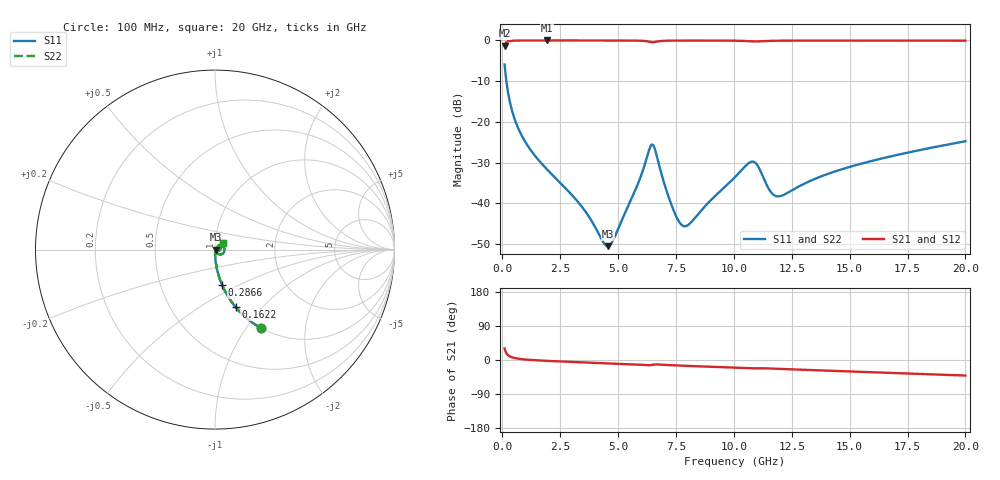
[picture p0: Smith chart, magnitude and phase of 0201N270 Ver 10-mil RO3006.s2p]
# GHz S MA R 50
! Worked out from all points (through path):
!   1601 points, 100 MHz to 20 GHz, reference 50 ohm
!   highest |S21| = -0.02 dB at 1.916 GHz (marker M1); lowest = -1.3 dB at 100 MHz (marker M2)
!   group delay of S21, straight-line fit = 6.12 ps
!   lowest |S11| = -50.5 dB at 4.553 GHz (marker M3), VSWR 1.01, Z = 50.3 - j0.0779 ohm
!   |S11| at or under -10 dB: 176 MHz to end of sweep
!   |S22| runs from -50.5 to -5.9 dB; largest |S21 - S12| = 0
!   S11 on the Smith chart (normalised r, x): 100 MHz: 1.00, -1.17; 162.2 MHz: 1.00, -0.72; 286.6 MHz: 1.00, -0.41; 20 GHz: 1.09, +0.09
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0.1  0.5062 -59.7  0.8616 30.2  0.8616 30.2  0.5062 -59.7
0.1621875  0.3402 -70.3  0.9396 19.6  0.9396 19.6  0.3402 -70.3
0.2865625  0.2002 -78.8  0.9789 11.0  0.9789 11.0  0.2002 -78.8
0.5104375  0.1132 -84.0  0.9926 5.5  0.9926 5.5  0.1132 -84.0
0.8338125  0.06847 -86.7  0.9965 2.3  0.9965 2.3  0.06847 -86.7
1.915875  0.02646 -88.5  0.9979 -2.2  0.9979 -2.2  0.02646 -88.5
3.420812  0.009244 -81.3  0.9975 -6.1  0.9975 -6.1  0.009244 -81.3
4.552625  0.002997 -15.0  0.9969 -8.8  0.9969 -8.8  0.002997 -15.0
4.801375  0.003619 18.4  0.9967 -9.4  0.9967 -9.4  0.003619 18.4
5.709313  0.01383 53.2  0.9939 -11.8  0.9939 -11.8  0.01383 53.2
6.405812  0.05054 10.4  0.9534 -13.6  0.9534 -13.6  0.05054 10.4
6.542625  0.05046 -21.7  0.95 -12.2  0.95 -12.2  0.05046 -21.7
6.741625  0.032 -51.8  0.9751 -11.8  0.9751 -11.8  0.032 -51.8
7.388375  0.008373 -51.3  0.9931 -14.0  0.9931 -14.0  0.008373 -51.3
7.848562  0.005265 -10.4  0.9946 -15.2  0.9946 -15.2  0.005265 -10.4
10.05  0.02108 45.6  0.991 -20.4  0.991 -20.4  0.02108 45.6
10.87087  0.03235 9.7  0.972 -21.9  0.972 -21.9  0.03235 9.7
11.57981  0.01405 -4.3  0.9863 -22.5  0.9863 -22.5  0.01405 -4.3
11.90319  0.01222 14.6  0.99 -23.3  0.99 -23.3  0.01222 14.6
13.37081  0.01932 45.5  0.9936 -26.6  0.9936 -26.6  0.01932 45.5
16.69162  0.03733 47.5  0.9933 -33.8  0.9933 -33.8  0.03733 47.5
20  0.05794 42.9  0.9918 -41.0  0.9918 -41.0  0.05794 42.9
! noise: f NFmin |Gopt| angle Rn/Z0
0.1  0.0005833  0.9266  0.2918  0.001764
2.301  0.004141  0.7803  4.498  0.003857
4.515  0.007244  0.7572  8.743  0.006002
6.729  0.02615  0.8924  13.01  0.05228
8.943  0.01332  0.7426  17.21  0.01015
11.14  0.03279  0.8616  21.4  0.04905
13.36  0.0176  0.7169  25.5  0.01171
15.57  0.01836  0.6907  29.54  0.01083
17.79  0.01993  0.6795  33.53  0.01106
20  0.02167  0.6728  37.46  0.01149
